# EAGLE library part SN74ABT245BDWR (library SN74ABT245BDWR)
Texas Instruments SN74ABT245BDWR, Bus Transceiver, 8-Bit Non-Inverting TTL, 5V, 20-Pin SOIC Source: Datasheet
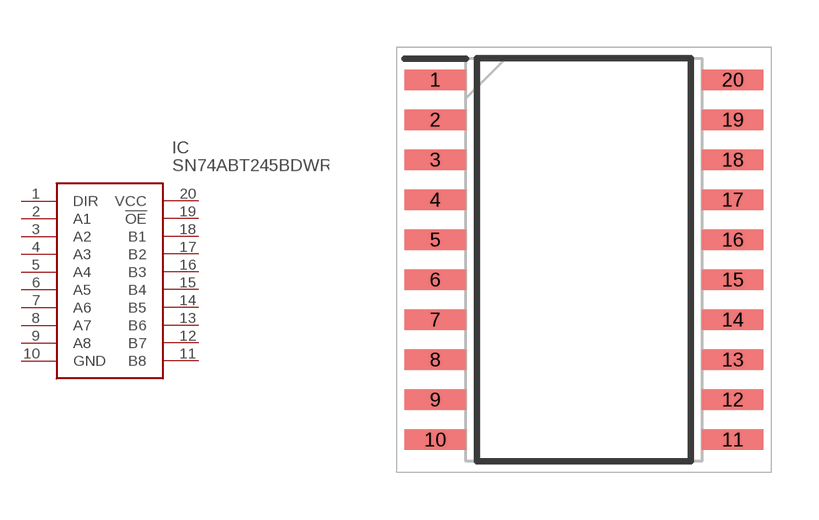
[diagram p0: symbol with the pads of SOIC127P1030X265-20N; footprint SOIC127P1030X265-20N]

Designator prefix IC

## SN74ABT245BDWR (Description: Texas Instruments SN74ABT245BDWR, Bus Transceiver, 8-Bit Non-Inverting TTL, 5V, 20-Pin SOIC; Height: 2.65mm; Manufacturer_Name: Texas Instruments; Manufacturer_Part_Number: SN74ABT245BDWR; Mouser_Part_Number: 595-SN74ABT245BDWR; Mouser_Price-Stock: https://www.mouser.co.uk/ProductDetail/Texas-Instruments/SN74ABT245BDWR?qs=afYny40WCj1jrBby8G5Ixw%3D%3D)  [SOIC127P1030X265-20N]
1  DIR
2  A1
3  A2
4  A3
5  A4
6  A5
7  A6
8  A7
9  A8
10  GND
11  B8
12  B7
13  B6
14  B5
15  B4
16  B3
17  B2
18  B1
19  !OE
20  VCC

## Footprint SOIC127P1030X265-20N (pad centres in mm)
DW (R-PDSO-G20)
smd 1.95 x 0.65: 1 -4.725,5.715; 2 -4.725,4.445; 3 -4.725,3.175; 4 -4.725,1.905; 5 -4.725,0.635; 6 -4.725,-0.635; 7 -4.725,-1.905; 8 -4.725,-3.175; 9 -4.725,-4.445; 10 -4.725,-5.715; 11 4.725,-5.715; 12 4.725,-4.445; 13 4.725,-3.175; 14 4.725,-1.905; 15 4.725,-0.635; 16 4.725,0.635; 17 4.725,1.905; 18 4.725,3.175; 19 4.725,4.445; 20 4.725,5.715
